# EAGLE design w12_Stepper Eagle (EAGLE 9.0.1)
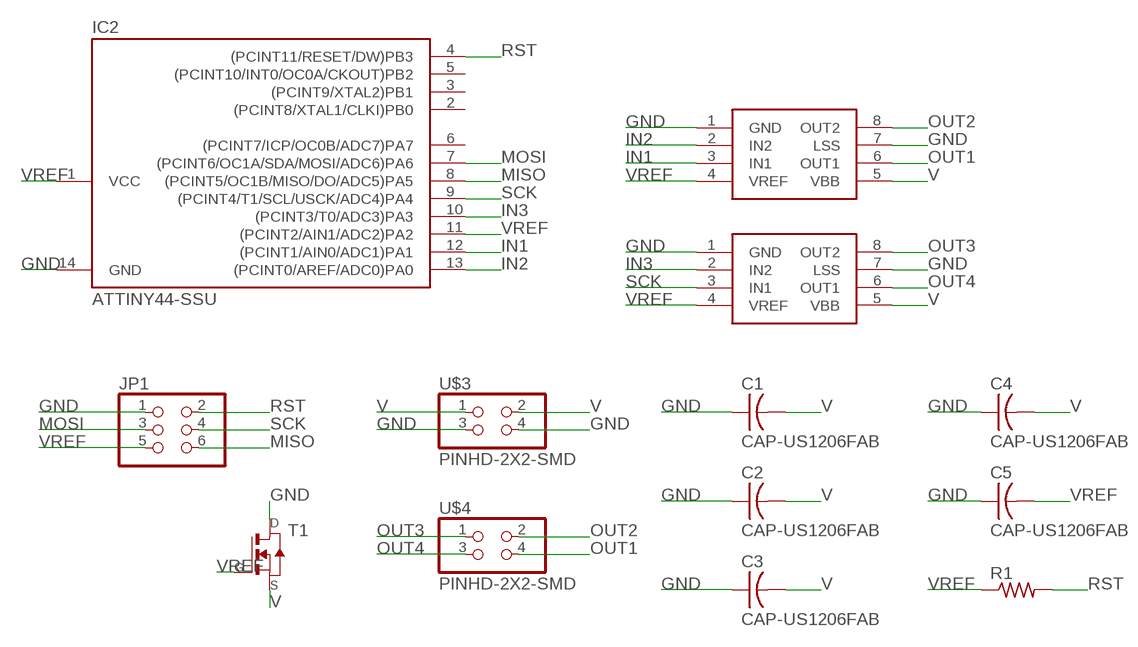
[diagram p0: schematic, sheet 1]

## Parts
C1  CAP-US1206FAB  [C1206FAB]
C2  CAP-US1206FAB  [C1206FAB]
C3  CAP-US1206FAB  [C1206FAB]
C4  CAP-US1206FAB  [C1206FAB]
C5  CAP-US1206FAB  [C1206FAB]
IC2  ATTINY44-SSU  [SOIC14]
JP1  PINHD-2X3-SMD  [2X03SMD]
R1  RES-US1206FAB  [R1206FAB]
T1  NMOSFETSOT23  [SOT-23]
U$1  A4953-H-BRIDGE-MOTOR-DRIVER  [SOIC8]
U$2  A4953-H-BRIDGE-MOTOR-DRIVER  [SOIC8]
U$3  PINHD-2X2-SMD  [2X02SMD]
U$4  PINHD-2X2-SMD  [2X02SMD]

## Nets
GND: C1.1 C2.1 C3.1 C4.1 C5.1 IC2.14(GND) JP1.1 T1.1(D) U$1.1(GND) U$1.7(LSS) U$2.1(GND) U$2.7(LSS) U$3.3 U$3.4
IN1: IC2.12((PCINT1/AIN0/ADC1)PA1) U$1.3(IN1)
IN2: IC2.13((PCINT0/AREF/ADC0)PA0) U$1.2(IN2)
IN3: IC2.10((PCINT3/T0/ADC3)PA3) U$2.2(IN2)
MISO: IC2.8((PCINT5/OC1B/MISO/DO/ADC5)PA5) JP1.6
MOSI: IC2.7((PCINT6/OC1A/SDA/MOSI/ADC6)PA6) JP1.3
OUT1: U$1.6(OUT1) U$4.4
OUT2: U$1.8(OUT2) U$4.2
OUT3: U$2.8(OUT2) U$4.1
OUT4: U$2.6(OUT1) U$4.3
RST: IC2.4((PCINT11/RESET/DW)PB3) JP1.2 R1.2
SCK: IC2.9((PCINT4/T1/SCL/USCK/ADC4)PA4) JP1.4 U$2.3(IN1)
V: C1.2 C2.2 C3.2 C4.2 T1.2(S) U$1.5(VBB) U$2.5(VBB) U$3.1 U$3.2
VREF: C5.2 IC2.1(VCC) IC2.11((PCINT2/AIN1/ADC2)PA2) JP1.5 R1.1 T1.3(G) U$1.4(VREF) U$2.4(VREF)
Unconnected: IC2.2((PCINT8/XTAL1/CLKI)PB0) IC2.3((PCINT9/XTAL2)PB1) IC2.5((PCINT10/INT0/OC0A/CKOUT)PB2) IC2.6((PCINT7/ICP/OC0B/ADC7)PA7)

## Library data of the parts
C1-C5 = fab:CAP-US
IC2 = fab:ATTINY44
JP1 = fab:PINHD-2X3-SMD: PIN HEADER
R1 = fab:RES-US: Resistor (US Symbol)
T1 = fab:NMOSFET: MOS FET
U$1 U$2 = fab:A4953-H-BRIDGE-MOTOR-DRIVER
U$3 U$4 = fab:PINHD-2X2-SMD

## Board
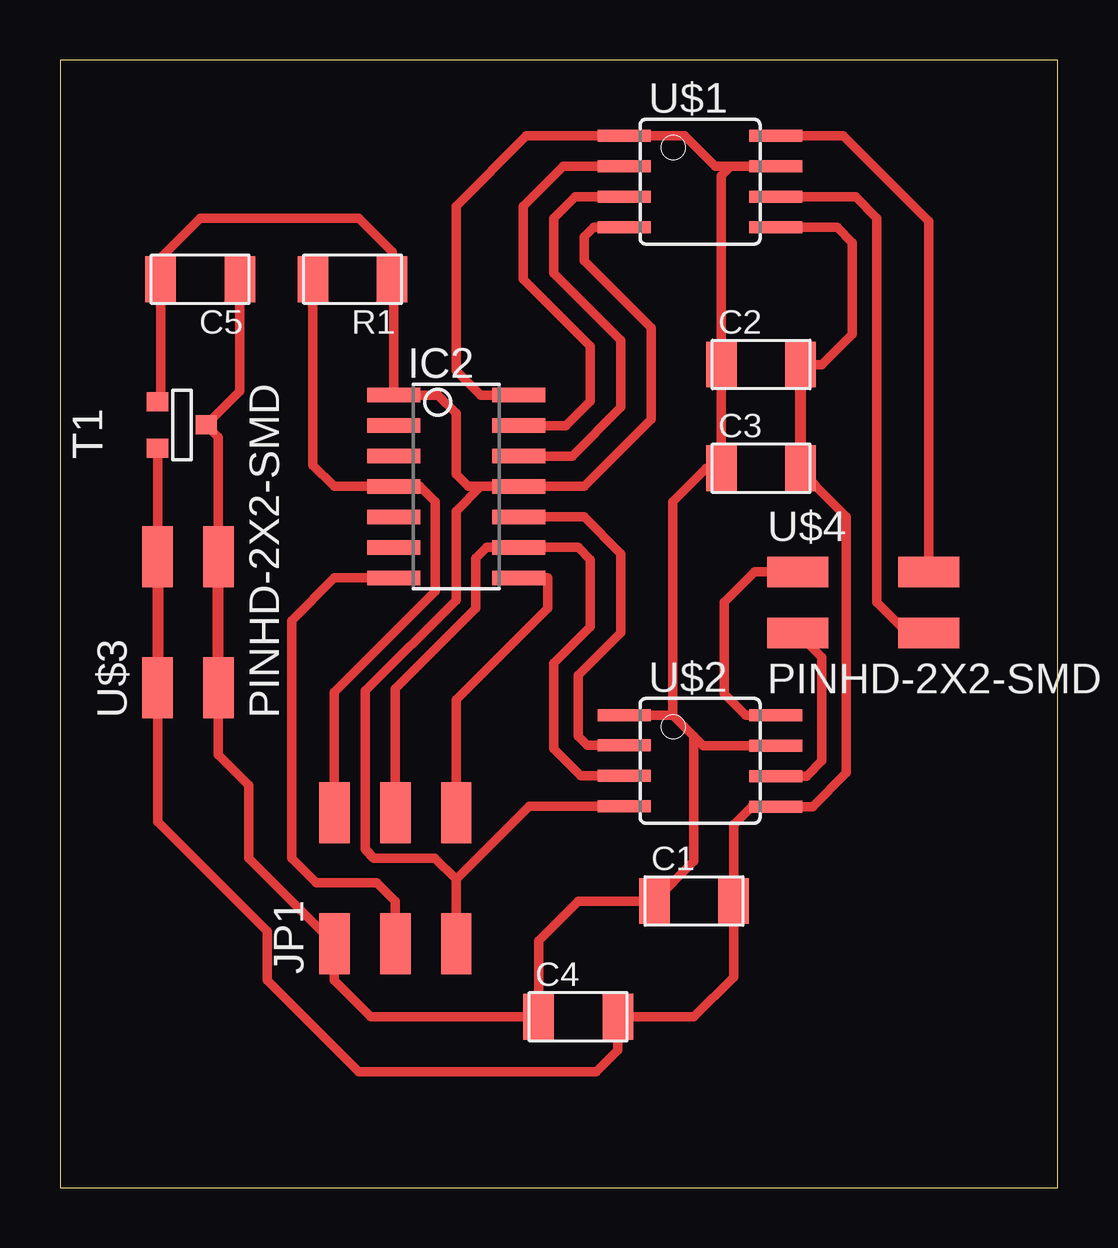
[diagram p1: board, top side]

Size 41.58 x 46.98 mm. Coordinates in mm from the lower left corner, seen from the top.
Outline: 0,0 41.58,0 41.58,46.98 0,46.98 0,0
Copper layers (1*16): Top 0.035mm / dielectric 1.5mm / Bottom 0.035mm
Design rules "IMP": minimum track width 0.45mm, minimum drill 0.35mm, track to track 0.42mm, track to pad 0.42mm, pad to pad 0.42mm, via to via 0.42mm, smd to smd 0.42mm, copper to edge 0.45mm, drill to drill 0.45mm, minimum pad ring 10mil, minimum via ring 8mil, stop-mask expansion 4mil, vias tented up to drill 0mil, thermal gap 10mil

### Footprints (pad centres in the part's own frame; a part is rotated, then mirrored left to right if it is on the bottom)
C1206FAB = smd 1.27 x 1.905: 1 -1.651,0; 2 1.651,0
SOIC14 = smd 0.61 x 2.21: 1 -3.81,-2.603; 2 -2.54,-2.603; 3 -1.27,-2.603; 4 0,-2.603; 5 1.27,-2.603; 6 2.54,-2.603; 7 3.81,-2.603; 8 3.81,2.603; 9 2.54,2.603; 10 1.27,2.603; 11 0,2.603; 12 -1.27,2.603; 13 -2.54,2.603; 14 -3.81,2.603
2X03SMD = smd 2.54 x 1.27: 1 -2.54,2.54; 2 2.92,2.54; 3 -2.54,0; 4 2.92,0; 5 -2.54,-2.54; 6 2.92,-2.54
R1206FAB = smd 1.27 x 1.905: 1 -1.651,0; 2 1.651,0
SOT-23 = smd 0.787 x 0.889: 1 0.025,-1.016; 2 -0.94,1.016; 3 0.991,1.016
SOIC8 = smd 0.5 x 2.2: 1 -1.905,-3.154; 2 -0.645,-3.154; 3 0.625,-3.154; 4 1.895,-3.154; 5 1.905,3.154; 6 0.635,3.154; 7 -0.635,3.154; 8 -1.905,3.154
2X02SMD = smd 2.54 x 1.27: 1 -2.54,1.27; 2 2.92,1.27; 3 -2.54,-1.27; 4 2.92,-1.27

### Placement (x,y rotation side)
C1  26.42,11.94 0 top
C2  29.21,34.29 0 top
C3  29.21,29.97 0 top
C4  21.59,7.11 0 top
C5  5.84,37.85 180 top
IC2  16.51,29.21 270 top
JP1  13.97,12.7 90 top
R1  12.19,37.85 180 top
T1  5.08,31.75 90 top
U$1  26.67,41.91 270 top
U$2  26.67,17.78 270 top
U$3  5.33,23.37 90 top
U$4  33.27,24.38 0 top

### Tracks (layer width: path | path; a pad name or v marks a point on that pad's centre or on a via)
GND
  Top 0.4: 27.94,42.55 27.3,42.55 26.04,43.81 U$1.1 19.43,43.81 16.51,40.89 16.51,34.04 17.53,33.02 IC2.14 | 27.94,42.55 U$1.7 | 27.94,42.55 27.56,42.16 C2.1 C3.1 26.92,29.97 25.53,28.57 25.53,19.69 | U$3.3 6.6,18.03 7.87,16.76 7.87,13.72 JP1.1 11.43,8.64 12.95,7.11 C4.1 19.94,10.29 21.59,11.94 C1.1 26.42,13.59 26.42,18.8 | U$3.4 6.6,31.27 T1.1 7.49,33.17 C5.1 | U$2.1 25.53,19.69 | 25.53,19.69 26.42,18.8 | U$2.7 26.8,18.41 26.42,18.8
  Top 0.45: U$3.3 U$3.4
IN1
  Top 0.4: IC2.12 21.34,30.48 23.37,32.51 23.37,35.31 20.57,38.1 20.57,40.39 21.47,41.28 U$1.3
IN2
  Top 0.4: IC2.13 21.08,31.75 22.1,32.77 22.1,35.05 19.3,37.85 19.3,40.89 20.96,42.55 U$1.2
IN3
  Top 0.4: U$2.2 21.96,18.42 21.59,18.8 21.59,21.34 23.37,23.11 23.37,26.42 21.84,27.94 IC2.10
MISO
  Top 0.4: JP1.6 16.51,20.32 20.32,24.13 20.32,25.4 IC2.8
MOSI
  Top 0.4: JP1.3 13.97,11.94 13.21,12.7 10.67,12.7 9.65,13.72 9.65,23.62 11.43,25.4 IC2.7
OUT1
  Top 0.4: U$1.6 33.15,41.27 34.04,40.39 34.04,24.38 35.31,23.11 U$4.4
OUT2
  Top 0.4: U$4.2 36.19,40.26 32.64,43.81 U$1.8
OUT3
  Top 0.4: U$2.8 28.57,19.69 27.69,20.57 27.69,24.38 28.96,25.65 U$4.1
OUT4
  Top 0.4: U$2.6 31.12,17.14 31.75,17.78 31.75,22.1 U$4.3
RST
  Top 0.4: JP1.2 11.43,20.64 15.63,24.84 15.63,28.56 14.99,29.21 IC2.4 11.43,29.21 10.54,30.1 R1.2
SCK
  Top 0.4: JP1.4 13.97,20.79 17.32,24.14 17.32,26.21 17.78,26.67 IC2.9 21.59,26.67 22.1,26.16 22.1,23.37 20.57,21.84 20.57,18.29 21.71,17.16 U$2.3
V
  Top 0.4: U$1.5 32.38,40 33.02,39.37 33.02,35.56 31.75,34.29 C2.2 | U$3.2 T1.2 | C3.2 31.5,29.21 32.77,27.94 32.77,17.27 31.37,15.88 U$2.5 28.83,15.88 28.07,15.11 C1.2 28.07,8.76 26.42,7.11 C4.2 23.24,5.71 22.35,4.83 12.45,4.83 8.64,8.64 8.64,10.67 4.06,15.24 U$3.1
  Top 0.45: U$3.2 U$3.1 | C3.2 C2.2
VREF
  Top 0.4: T1.3 4.19,32.87 C5.2 4.19,38.73 5.84,40.39 12.45,40.39 13.84,38.99 R1.1 13.91,37.78 IC2.1 15.75,33.02 16.51,32.26 16.51,29.72 17.02,29.21 17.53,29.21 | 17.53,29.21 IC2.11 21.84,29.21 24.64,32 24.64,35.81 21.84,38.61 21.84,39.62 22.23,40.02 U$1.4 | JP1.5 16.51,12.84 | 17.53,29.21 16.5,28.19 16.5,24.48 12.71,20.69 12.71,14.09 13.08,13.73 15.62,13.73 16.51,12.84 | 16.51,12.84 19.56,15.88 U$2.4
